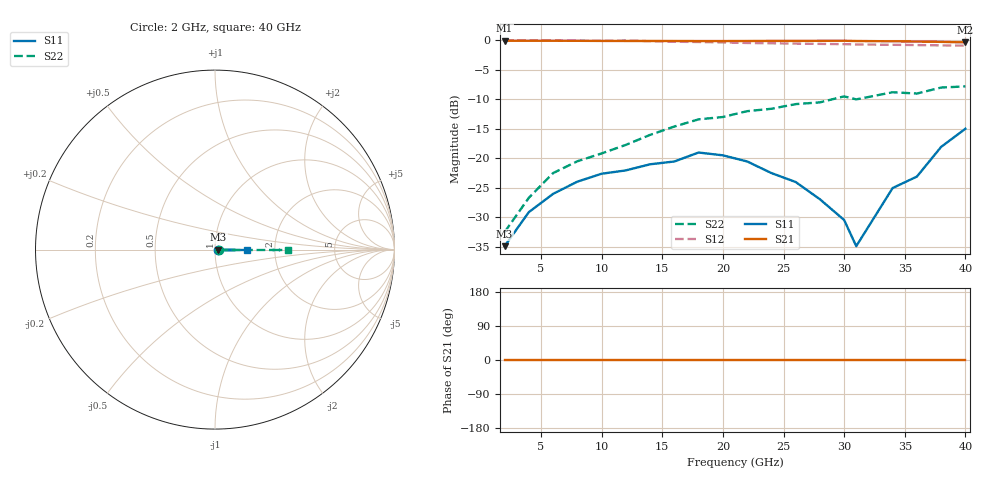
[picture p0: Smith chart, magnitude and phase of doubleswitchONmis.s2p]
# GHZ S MA R 50
!Output file by Shape3_28
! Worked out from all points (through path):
!   20 points, 2 GHz to 40 GHz, reference 50 ohm
!   highest |S21| = -0.05 dB at 2 GHz (marker M1); lowest = -0.4 dB at 40 GHz (marker M2)
!   lowest |S11| = -34.9 dB at 2 GHz (marker M3), VSWR 1.04, Z = 51.8 + j0 ohm
!   |S11| at or under -10 dB: start of sweep to end of sweep
!   |S22| runs from -32.5 to -7.8 dB; largest |S21 - S12| = 0.065
2  0.018 0.0  0.994 0.0  0.9979 0.0  0.0237 0.0
4  0.035 0.0  0.993 0.0  0.9972 0.0  0.0463 0.0
6  0.05 0.0  0.992 0.0  0.9951 0.0  0.075 0.0
8  0.0634 0.0  0.991 0.0  0.9934 0.0  0.0944 0.0
10  0.074 0.0  0.989 0.0  0.9917 0.0  0.11 0.0
12  0.079 0.0  0.988 0.0  0.9965 0.0  0.13 0.0
14  0.089 0.0  0.988 0.0  0.983 0.0  0.158 0.0
16  0.094 0.0  0.987 0.0  0.973 0.0  0.186 0.0
18  0.112 0.0  0.986 0.0  0.968 0.0  0.214 0.0
20  0.106 0.0  0.986 0.0  0.96 0.0  0.224 0.0
22  0.0941 0.0  0.987 0.0  0.95 0.0  0.251 0.0
24  0.075 0.0  0.989 0.0  0.944 0.0  0.263 0.0
26  0.063 0.0  0.989 0.0  0.938 0.0  0.288 0.0
28  0.045 0.0  0.991 0.0  0.9332 0.0  0.298 0.0
30  0.03 0.0  0.992 0.0  0.9279 0.0  0.335 0.0
31  0.018 0.0  0.987 0.0  0.9225 0.0  0.316 0.0
34  0.056 0.0  0.982 0.0  0.917 0.0  0.363 0.0
36  0.07 0.0  0.977 0.0  0.912 0.0  0.354 0.0
38  0.125 0.0  0.971 0.0  0.906 0.0  0.398 0.0
40  0.178 0.0  0.96 0.0  0.902 0.0  0.407 0.0
